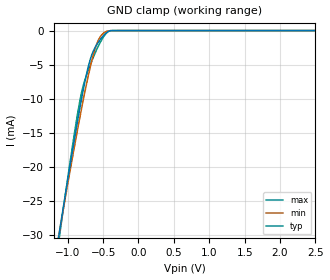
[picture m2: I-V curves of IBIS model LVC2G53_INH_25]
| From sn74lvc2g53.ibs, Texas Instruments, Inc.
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[Model]   LVC2G53_INH_25
Model_type  Input
Vinl=0.7
Vinh=1.7
| variable   typ   min   max
C_comp   3.37pF   2.85pF   4.09pF
[Temperature Range]   40   100   -40
| Ambient temperature   25   85   -40
[Voltage range]   2.5   2.3   2.7
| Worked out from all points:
|   GND clamp passes 1 mA (typ) near -0.52 V on its own axis
[GND Clamp]
| LVC2G53_INH_25
|   Voltage   I(typ)   I(min)   I(max)
-5.5V     -348.1mA   -320.8mA   -389.9mA
-1.145V   -31.41mA   -31.26mA   -32.35mA
-1.105V   -28.77mA   -28.83mA   -29.37mA
-895mV    -15.37mA   -16.48mA   -14.42mA
-840mV    -12.09mA   -13.41mA   -10.99mA
-790mV    -9.266mA   -10.72mA   -8.474mA
-690mV    -4.56mA    -5.755mA   -5.288mA
-645mV    -3.18mA    -3.843mA   -4.107mA
-600mV    -2.253mA   -2.277mA   -3.017mA
-525mV    -1.127mA   -702uA     -1.455mA
-435mV    -182.9uA   -61.02uA   -202.3uA
2.5V      145.8pA    548.3pA    1.222nA
